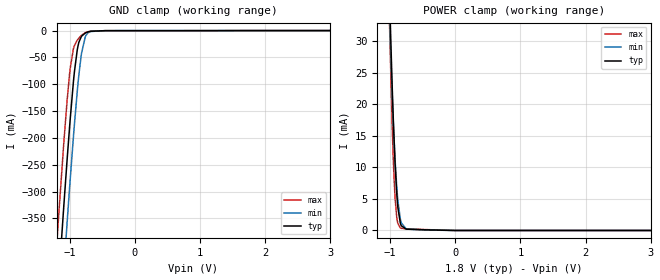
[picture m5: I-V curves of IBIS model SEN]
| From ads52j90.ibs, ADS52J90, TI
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|   Model
[Model]   SEN
Model_type   Input
Vinl = 0.45
Vinh = 1.35
|   typ   min   max
C_comp   1.431pF   1.417pF   1.444pF
[Voltage Range]   1.8   1.7   1.9
[Temperature Range]   25   85   -40
[Power Clamp Reference]   1.8   1.7   1.9
[GND Clamp Reference]   -0   -0   -0
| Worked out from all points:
|   GND clamp passes 1 mA (typ) near -0.61 V on its own axis
|   POWER clamp passes 1 mA (typ) near -0.84 V on its own axis
[GND Clamp]
|   Voltage   I(typ)   I(min)   I(max)
-1.8V     -1.671A    -1.791A    -1.551A
-1.195V   -518.1mA   -640mA     -395.6mA
-1.174V   -478.7mA   -600.4mA   -356.7mA
-1.087V   -325.1mA   -444.8mA   -207.5mA
-1.039V   -242.5mA   -359.8mA   -131.9mA
-990mV    -165.1mA   -277.6mA   -70.38mA
-941.4mV  -96.51mA   -199.5mA   -34.43mA
-882mV    -36.3mA    -113.7mA   -18.02mA
-817.2mV  -10.64mA   -42.92mA   -8.983mA
-757.8mV  -4.39mA    -11.3mA    -4.002mA
-450mV    -158.3uA   -103.7uA   -240.5uA
3.595V    0A         0A         0A
[POWER Clamp]
|   Voltage   I(typ)   I(min)   I(max)
-1.8V     409.9mA    346.5mA    478.7mA
-1.012V   37.77mA    33.77mA    33.5mA
-1.006V   35.75mA    32.11mA    31.14mA
-973.8mV  24.36mA    22.75mA    18.26mA
-957.6mV  19.26mA    18.53mA    12.88mA
-925.2mV  10.72mA    11.31mA    5.146mA
-898.2mV  5.679mA    6.758mA    1.969mA
-882mV    3.638mA    4.73mA     1.104mA
-844.2mV  1.167mA    1.838mA    418.2uA
-752.4mV  208.5uA    227.2uA    251.6uA
-450mV    101.6uA    72.86uA    140.7uA
3.595V    0A         0A         0A
